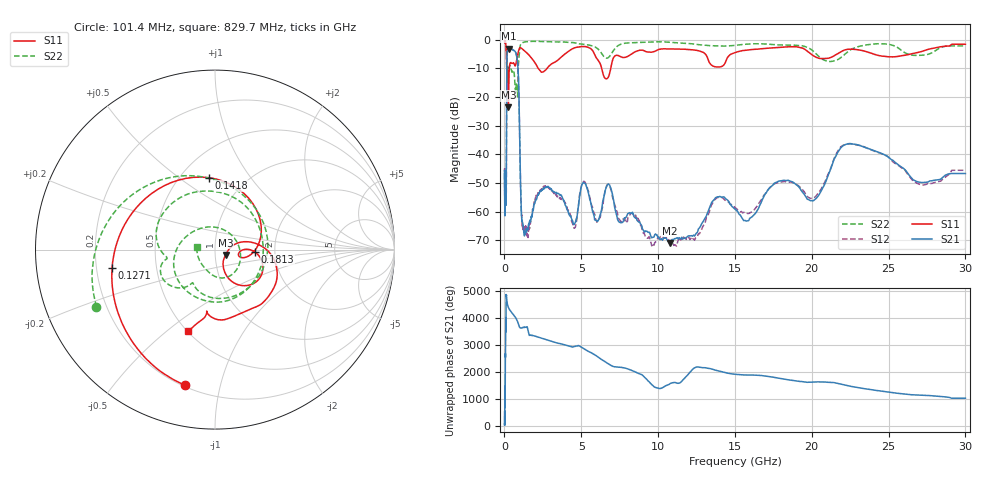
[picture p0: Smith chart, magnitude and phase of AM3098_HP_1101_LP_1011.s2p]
! Date/Time: Thu, Feb 28, 2019 8:45 AM
! Network Analyzer: Agilent Technologies E8364B Rev: A.07.50.67
! Sweep from 0.010 to 30.000 GHz, 1601 Points, Sweep Type: LOG
! Power Supply: 5.022 V, 0.002 A
# Hz S DB R 50
!freq MagS11 AngS11 MagS21 AngS21 MagS12 AngS12 MagS22 AngS22
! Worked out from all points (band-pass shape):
!   1601 points, 10 MHz to 30 GHz, reference 50 ohm
!   highest |S21| = -3.11 dB at 266.5 MHz (marker M1); lowest = -71.0 dB at 10.76 GHz (marker M2)
!   |S21| within 3 dB of the highest: 159.3 MHz to 806.5 MHz (647.2 MHz wide, 134 % of centre)
!   lowest |S11| = -23.6 dB at 252.2 MHz (marker M3), VSWR 1.14, Z = 56.2 - j3.31 ohm
!   |S11| at or under -10 dB: 148 MHz to 318.3 MHz (170.3 MHz wide, 73.1 % of centre); 2.194 GHz to 2.779 GHz (585.2 MHz wide, 23.5 % of centre); 6.326 GHz to 6.918 GHz (592.6 MHz wide, 8.95 % of centre)
!   |S22| runs from -20.0 to -0.6 dB; largest |S21 - S12| = 0.009
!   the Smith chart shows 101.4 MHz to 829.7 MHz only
!   S11 on the Smith chart (normalised r, x): 101.4 MHz: 0.21, -0.78; 127.1 MHz: 0.27, -0.08; 141.8 MHz: 0.68, +0.65; 181.3 MHz: 1.57, -0.04; 829.7 MHz: 0.51, -0.60
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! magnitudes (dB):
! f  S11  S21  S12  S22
! 10 MHz  -0.3  -46.8  -46.1  -0.6
! 38.04 MHz  -0.3  -57.2  -57.3  -0.8
! 101.4 MHz  -2.2  -54.9  -53.5  -2.7
! 127.1 MHz  -4.7  -42.3  -42.6  -6.0
! 141.8 MHz  -7.9  -17.7  -17.7  -10.6
! 144.7 MHz  -8.8  -14.3  -14.3  -10.9
! 181.3 MHz  -13.1  -4.2  -4.2  -11.0
! 252.2 MHz  -23.6  -3.2  -3.1  -11.3
! 266.5 MHz  -19.6  -3.1  -3.1  -11.2
! 550.5 MHz  -8.2  -3.6  -3.6  -10.8
! 829.7 MHz  -6.4  -6.9  -6.9  -20.0
! 921.7 MHz  -3.9  -15.0  -14.9  -7.6
! 1.071 GHz  -2.9  -55.8  -55.6  -1.5
! 1.184 GHz  -3.4  -64.0  -65.5  -1.0
! 2.084 GHz  -9.0  -55.7  -54.2  -0.6
! 4.525 GHz  -3.0  -64.5  -65.8  -1.1
! 5.18 GHz  -2.4  -50.0  -49.5  -1.7
! 7.926 GHz  -6.1  -61.9  -62.7  -1.2
! 10.76 GHz  -3.3  -71.0  -70.5  -1.0
! 20.1 GHz  -5.6  -56.3  -55.3  -4.1
! 22.56 GHz  -3.4  -36.3  -36.4  -3.5
! 30 GHz  -1.6  -46.7  -45.6  -2.2
